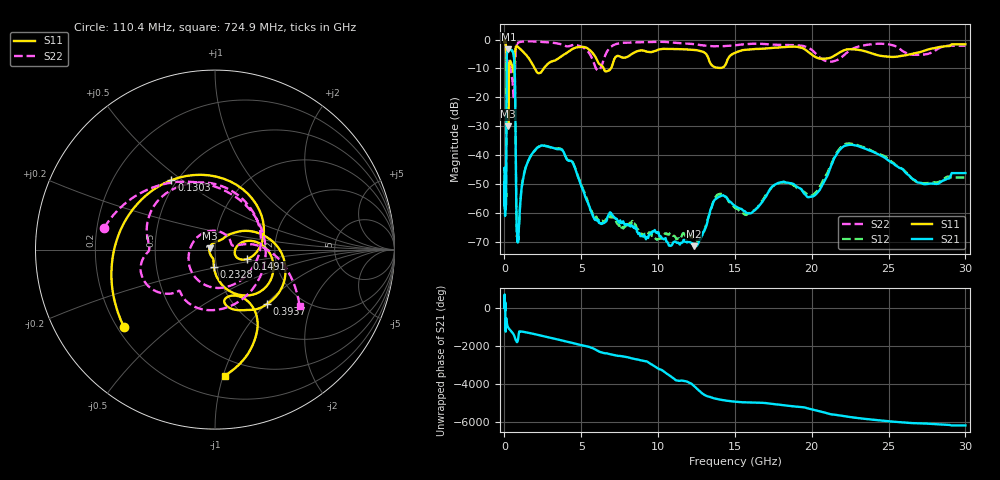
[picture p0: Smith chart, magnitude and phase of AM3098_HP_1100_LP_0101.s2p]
! Date/Time: Thu, Feb 28, 2019 8:44 AM
! Network Analyzer: Agilent Technologies E8364B Rev: A.07.50.67
! Sweep from 0.010 to 30.000 GHz, 1601 Points, Sweep Type: LOG
! Power Supply: 5.023 V, 0.002 A
# Hz S DB R 50
!freq MagS11 AngS11 MagS21 AngS21 MagS12 AngS12 MagS22 AngS22
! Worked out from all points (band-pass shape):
!   1601 points, 10 MHz to 30 GHz, reference 50 ohm
!   highest |S21| = -3.39 dB at 262.5 MHz (marker M1); lowest = -71.5 dB at 12.31 GHz (marker M2)
!   |S21| within 3 dB of the highest: 148.5 MHz to 623.5 MHz (474.9 MHz wide, 123 % of centre)
!   lowest |S11| = -30.0 dB at 246 MHz (marker M3), VSWR 1.07, Z = 47 + j0.768 ohm
!   |S11| at or under -10 dB: 205.2 MHz to 298.4 MHz (93.1 MHz wide, 37 % of centre); 1.974 GHz to 2.552 GHz (578.4 MHz wide, 25.6 % of centre); 6.463 GHz to 6.931 GHz (467.9 MHz wide, 6.99 % of centre)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
!   |S22| runs from -20.3 to -0.6 dB; largest |S21 - S12| = 0.011
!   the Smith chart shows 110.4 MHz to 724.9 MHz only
!   S11 on the Smith chart (normalised r, x): 110.4 MHz: 0.23, -0.35; 130.3 MHz: 0.47, +0.46; 149.1 MHz: 1.43, -0.15; 232.8 MHz: 0.97, -0.19; 393.7 MHz: 1.38, -1.02; 724.9 MHz: 0.36, -1.01
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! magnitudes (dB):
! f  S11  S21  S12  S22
! 10 MHz  -0.4  -44.8  -46.4  -0.6
! 38.04 MHz  -0.4  -58.8  -57.3  -0.8
! 110.4 MHz  -3.5  -49.9  -50.7  -4.0
! 130.3 MHz  -6.8  -20.4  -20.5  -10.9
! 144.7 MHz  -11.8  -7.6  -7.5  -9.5
! 149.1 MHz  -14.6  -6.3  -6.2  -10.0
! 198.3 MHz  -9.2  -4.0  -4.0  -7.3
! 232.8 MHz  -20.2  -3.5  -3.5  -8.6
! 246 MHz  -30.0  -3.4  -3.4  -8.7
! 262.5 MHz  -18.4  -3.4  -3.4  -8.6
! 393.7 MHz  -7.5  -3.6  -3.6  -9.3
! 550.5 MHz  -10.7  -4.4  -4.3  -16.8
! 659.1 MHz  -6.8  -9.6  -9.6  -15.6
! 724.9 MHz  -3.0  -33.1  -32.9  -5.0
! 789.2 MHz  -2.3  -63.3  -64.3  -1.9
! 868 MHz  -2.5  -68.9  -65.7  -1.2
! 2.084 GHz  -11.1  -37.7  -37.7  -0.7
! 3.723 GHz  -5.8  -38.1  -38.0  -1.7
! 7.926 GHz  -6.2  -63.9  -64.6  -1.1
! 12.31 GHz  -3.6  -71.5  -68.7  -1.6
! 22.56 GHz  -3.3  -36.4  -36.0  -3.5
! 30 GHz  -1.7  -46.2  -47.8  -2.1
